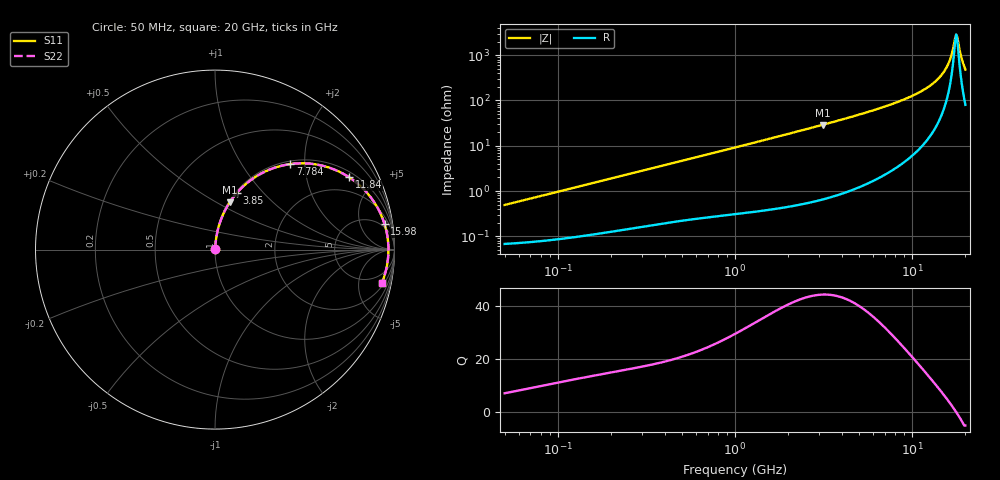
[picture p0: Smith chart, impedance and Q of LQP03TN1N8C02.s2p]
!Murata Part Number: LQP03TN1N8C02
!These Parameters are Measured in Series Mode Connection
!  o--[Z]--o
!Port1  Port2
!  o-------o
!Freq. Start=50[MHz] Stop=20[GHz], 401[Steps]
# Hz S RI R 50
!Freq.(Hz) S11(Real) S11(Imag) S21(Real) S21(Imag) S12(Real) S12(Imag) S22(Real) S22(Imag)
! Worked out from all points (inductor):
!   401 points, 50 MHz to 20 GHz, reference 50 ohm
!   read as one part in series: L = 1.55 nH near 51.52 MHz
!   highest Q = 44.5 at 3.122 GHz (marker M1), where L = 1.48 nH
!   self-resonance near 17.74 GHz
!   S11 on the Smith chart (normalised r, x): 50 MHz: 1.00, +0.01; 3.85 GHz: 1.02, +0.72; 7.784 GHz: 1.06, +1.69; 11.84 GHz: 1.23, +3.57; 15.98 GHz: 4, +12; 20 GHz: 2.60, -9.49
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5e7  0.000704 0.00488  0.9993 -0.00488  0.9993 -0.00488  0.000704 0.00488
1.364002e8  0.00118 0.0131  0.9988 -0.0131  0.9988 -0.0131  0.00118 0.0131
3.721004e8  0.00306 0.0346  0.9969 -0.0346  0.9969 -0.0346  0.00306 0.0346
1e9  0.0113 0.0901  0.9887 -0.0901  0.9887 -0.0901  0.0113 0.0901
2.728004e9  0.0642 0.2339  0.9358 -0.2339  0.9358 -0.2339  0.0642 0.2339
3.121702e9  0.0823 0.2639  0.9177 -0.2639  0.9177 -0.2639  0.0823 0.2639
3.850025e9  0.1214 0.3154  0.8786 -0.3154  0.8786 -0.3154  0.1214 0.3154
5.433528e9  0.2274 0.4064  0.7726 -0.4064  0.7726 -0.4064  0.2274 0.4064
7.442007e9  0.39 0.4715  0.61 -0.4715  0.61 -0.4715  0.39 0.4715
7.784049e9  0.4193 0.4765  0.5807 -0.4765  0.5807 -0.4765  0.4193 0.4765
9.745021e9  0.5869 0.47  0.4131 -0.47  0.4131 -0.47  0.5869 0.47
1.183995e10  0.7481 0.4025  0.2519 -0.4025  0.2519 -0.4025  0.7481 0.4025
1.417136e10  0.8827 0.2705  0.1173 -0.2705  0.1173 -0.2705  0.8827 0.2705
1.504638e10  0.9177 0.2101  0.0823 -0.2101  0.0823 -0.2101  0.9177 0.2101
1.597544e10  0.9448 0.1416  0.0552 -0.1416  0.0552 -0.1416  0.9448 0.1416
1.646126e10  0.9547 0.1043  0.0453 -0.1043  0.0453 -0.1043  0.9547 0.1043
1.747767e10  0.9657 0.024  0.0343 -0.024  0.0343 -0.024  0.9657 0.024
1.774144e10  0.9663 0.00279  0.0337 -0.00279  0.0337 -0.00279  0.9663 0.00279
1.800918e10  0.966 -0.0189  0.034 0.0189  0.034 0.0189  0.966 -0.0189
1.828096e10  0.9647 -0.0411  0.0353 0.0411  0.0353 0.0411  0.9647 -0.0411
1.912117e10  0.9537 -0.1105  0.0463 0.1105  0.0463 0.1105  0.9537 -0.1105
2e10  0.9301 -0.1842  0.0699 0.1842  0.0699 0.1842  0.9301 -0.1842
